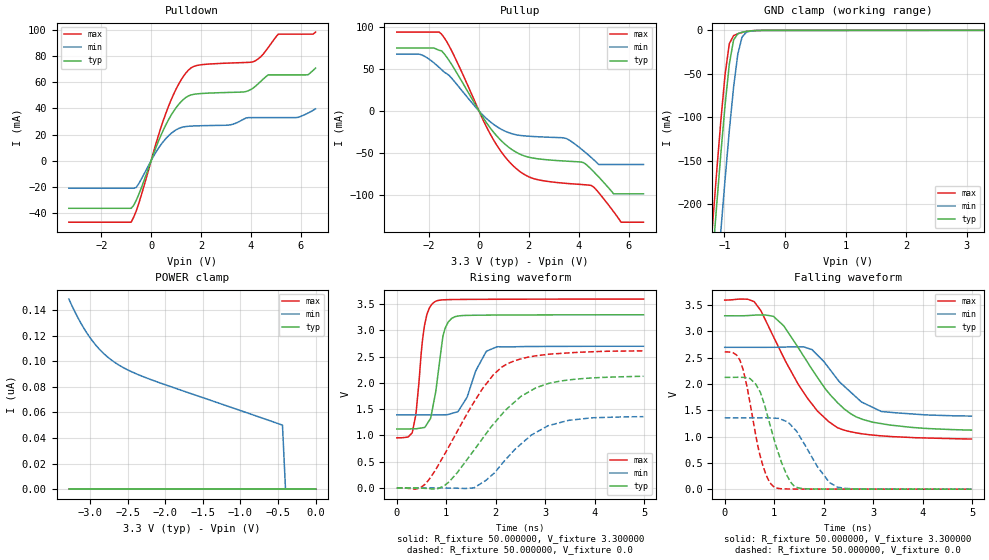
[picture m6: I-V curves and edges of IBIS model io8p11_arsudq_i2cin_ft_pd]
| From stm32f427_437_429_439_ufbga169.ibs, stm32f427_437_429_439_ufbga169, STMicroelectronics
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|   Model io8p11_arsudq_i2cin_ft_pd
[Model]  io8p11_arsudq_i2cin_ft_pd
Model_type I/O
Polarity   Non-Inverting
Enable   Active-Low
Vinl =   0.990000V
Vinh =   2.310000V
Vmeas =  1.650000V
Cref =   30.000000pF
Rref =   100.000000M
Vref =   0.0V
C_comp   2.280000pF   2.217100pF   2.355700pF
[Temperature Range]   25.000000   0.125000k   -40.000000
[Pullup Reference]   3.300000V   2.700000V   3.600000V
[Pulldown Reference]   0.0V   0.0V   0.0V
[POWER Clamp Reference]   3.300000V   2.700000V   3.600000V
[GND Clamp Reference]   0.0V   0.0V   0.0V
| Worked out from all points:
|   slope of the pulldown table from 0 to 0.495 V, typ, clamps not added: 20.9 ohm
|   slope of the pullup table from 0 to 0.495 V, typ, clamps not added: 22.6 ohm
|   GND clamp passes 1 mA (typ) near -0.62 V on its own axis
|   rising waveform, R_fixture 50.000000, V_fixture 3.300000: 20-80 % time 197ps typ, 344ps min, 161ps max; typ from 1.12 V to 3.3 V
|   rising waveform, R_fixture 50.000000, V_fixture 0.0: 20-80 % time 1.13ns typ, 913ps min, 1ns max; typ from 0 V to 2.13 V
|   falling waveform, R_fixture 50.000000, V_fixture 3.300000: 20-80 % time 1.01ns typ, 784ps min, 979ps max; typ from 3.3 V to 1.12 V
|   falling waveform, R_fixture 50.000000, V_fixture 0.0: 20-80 % time 414ps typ, 536ps min, 331ps max; typ from 2.13 V to 0 V
[Pulldown]
|Voltage   I(typ)   I(min)   I(max)
-3.3V     -36.46mA   -21.1mA    -47.09mA
-800mV    -36.46mA   -21.1mA    -47.09mA
-600mV    -30.5mA    -20.54mA   -38.69mA
700mV     31.4mA     19.11mA    41.71mA
1.2V      45.15mA    25.37mA    61.75mA
1.6V      50.35mA    26.5mA     71.06mA
3.1V      52.27mA    27.26mA    74.75mA
4.1V      55.7mA     32.99mA    75.8mA
4.7V      65.72mA    32.99mA    86.69mA
5.1V      65.72mA    32.99mA    96.9mA
6.3V      65.87mA    36.5mA     96.9mA
6.6V      70.93mA    39.71mA    98.5mA
[Pullup]
|Voltage   I(typ)   I(min)   I(max)
-3.3V     74.73mA    67.41mA    93.65mA
-2.3V     74.73mA    66.57mA    93.65mA
-1.5V     71.37mA    49.01mA    91.08mA
500mV     -22.07mA   -14mA      -30.03mA
1.6V      -50.64mA   -28.81mA   -70.96mA
3.5V      -59.53mA   -32.65mA   -85.92mA
4.2V      -61.43mA   -47.49mA   -87.46mA
4.5V      -69.06mA   -55.12mA   -88.38mA
4.8V      -78.22mA   -63.5mA    -96.84mA
5.4V      -98.3mA    -63.5mA    -119.6mA
5.7V      -98.3mA    -63.5mA    -132mA
6.6V      -98.3mA    -63.5mA    -132mA
[GND_clamp]
|Voltage   I(typ)   I(min)   I(max)
-3.3V     -2.315A    -2.395A    -2.287A
-1.2V     -265.5mA   -356.1mA   -227.2mA
-1.13V    -202.7mA   -292.9mA   -164.1mA
-1.06V    -142.2mA   -231.2mA   -104.1mA
-990mV    -85.98mA   -171.6mA   -50.73mA
-920mV    -38.81mA   -115.5mA   -15.29mA
-850mV    -11.09mA   -65.61mA   -6.016mA
-780mV    -3.793mA   -27.42mA   -3.89mA
-710mV    -2.098mA   -7.698mA   -2.396mA
-640mV    -1.159mA   -2.127mA   -1.234mA
-570mV    -535.1uA   -807.4uA   -490.2uA
3.28V     81.28uA    57.87uA    93.98uA
[POWER_clamp]
|Voltage   I(typ)   I(min)   I(max)
-3.28V    0A         148.5nA    0A
-3.2V     0A         138.6nA    0A
-3.12V    0A         129.7nA    0A
-3.04V    0A         122nA      0A
-2.96V    0A         115.3nA    0A
-2.8V     0A         105.1nA    0A
-2.6V     0A         96.44nA    0A
-2.4V     0A         90.52nA    0A
-2.16V    0A         84.97nA    0A
-440mV    0A         50.04nA    0A
-400mV    0A         0A         0A
0V        0A         0A         0A
[Ramp]
| variable   typ   min   max
dV/dt_r  1.26072/1.11586n   0.80532/0.90425n   1.56000/0.99961n
dV/dt_f  1.27662/0.99479n   0.77220/0.76589n   1.56944/0.97113n
R_load = 50.000000
[Rising Waveform]
R_fixture= 50.000000
V_fixture= 3.300000
V_fixture_min= 2.700000
V_fixture_max= 3.600000
|time   V(typ)   V(min)   V(max)
0s        1.123V     1.391V     954mV
310.3ps   1.125V     1.391V     1.048V
390.4ps   1.127V     1.391V     1.435V
560.6ps   1.152V     1.391V     3.098V
780.8ps   1.799V     1.39V      3.553V
951ps     2.96V      1.393V     3.584V
1.171ns   3.26V      1.435V     3.589V
1.802ns   3.292V     2.59V      3.593V
2.022ns   3.293V     2.688V     3.594V
4.985ns   3.299V     2.699V     3.598V
[Rising Waveform]
R_fixture= 50.000000
V_fixture= 0.0
V_fixture_min= 0.0
V_fixture_max= 0.0
|time   V(typ)   V(min)   V(max)
0s        345.5uV    196.9uV    641.9uV
470.5ps   -3.051mV   137.9uV    402.6uV
660.7ps   -15.09mV   184.1uV    170.3mV
951ps     36.13mV    -1.054mV   617.8mV
1.562ns   720.8mV    2.763mV    1.636V
1.952ns   1.214V     268.5mV    2.155V
2.202ns   1.487V     543.3mV    2.348V
2.713ns   1.854V     1.003V     2.501V
3.063ns   1.989V     1.186V     2.546V
4.985ns   2.127V     1.357V     2.611V
[Falling Waveform]
R_fixture= 50.000000
V_fixture= 3.300000
V_fixture_min= 2.700000
V_fixture_max= 3.600000
|time   V(typ)   V(min)   V(max)
0s        3.299V     2.699V     3.598V
590.6ps   3.31V      2.699V     3.569V
730.7ps   3.315V     2.699V     3.396V
991ps     3.282V     2.7V       2.891V
1.201ns   3.097V     2.704V     2.486V
1.762ns   2.283V     2.656V     1.622V
2.272ns   1.654V     2.098V     1.173V
2.653ns   1.377V     1.754V     1.072V
3.163ns   1.247V     1.478V     1.014V
4.985ns   1.123V     1.391V     954mV
[Falling Waveform]
R_fixture= 50.000000
V_fixture= 0.0
V_fixture_min= 0.0
V_fixture_max= 0.0
|time   V(typ)   V(min)   V(max)
0s        2.127V     1.357V     2.611V
310.3ps   2.128V     1.357V     2.448V
450.5ps   2.117V     1.357V     1.953V
630.6ps   1.993V     1.357V     1.01V
830.8ps   1.514V     1.359V     283.4mV
1.011ns   903.9mV    1.351V     37.26mV
1.391ns   70.22mV    1.164V     2.812mV
1.872ns   3.087mV    430.9mV    1.932mV
2.272ns   1.681mV    41.84mV    1.69mV
4.985ns   345.5uV    196.9uV    641.9uV
